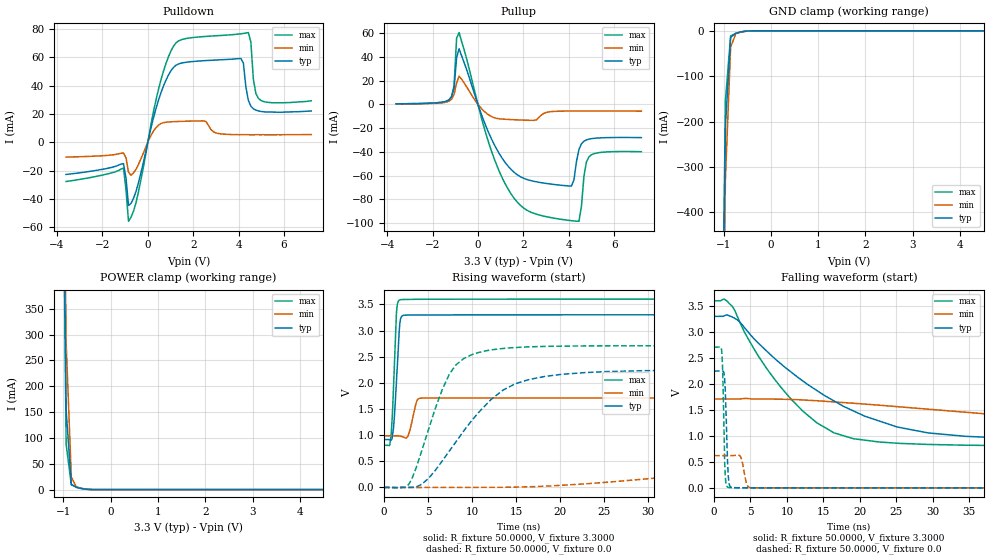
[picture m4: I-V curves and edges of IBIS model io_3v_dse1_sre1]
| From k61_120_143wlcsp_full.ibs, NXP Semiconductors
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[Model]  io_3v_dse1_sre1
|   Model io_3v_dse1_sre1
| Library cells for typ/min/max conditions are connected as defined below:
|  pad - External Pad
|  ipp_do_3v - Core Input
|  ipp_obe_3v - Output Buffer Enable
|  esd_boost - vdd_s_3v
|  esd_trigger - vss_s_3v
|  ipp_ame_3v - vss_s_3v
|  ipp_dse_3v - vdd_s_3v
|  ipp_ina_3v - NC
|  ipp_ina_mux_3v - NC
|  ipp_ind_3v - NC
|  ipp_pue_3v - vss_s_3v
|  ipp_sre_3v - vdd_s_3v
|  tie_3v - vdd_s_3v
|  tie_hi - vdd_s_lv
|  vbuf_3v - vdd_s_3v
|  vdd_s_3v - vdd_s_3v
|  vdd_s_lv - vdd_s_lv
|  vss_bulk - vss_s_3v
|  vss_s_3v - vss_s_3v
| All other pins connected to ground
Model_type I/O
Polarity   Non-Inverting
Enable   Active-High
Vinl =   1.1550V
Vinh =   2.3100V
Vmeas =  1.6500V
Cref =   25.0000pF
Rref =   50.0000
Vref =   0.0V
C_comp   1.9040pF   1.7928pF   2.1191pF
[Temperature Range]   25.0000   0.1250k   -40.0000
[Voltage Range]   3.3000V   1.7100V   3.6000V
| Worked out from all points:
|   slope of the pulldown table from 0 to 0.495 V, typ, clamps not added: 16 ohm
|   slope of the pullup table from 0 to 0.495 V, typ, clamps not added: 19.9 ohm
|   GND clamp passes 1 mA (typ) near -0.54 V on its own axis
|   POWER clamp passes 1 mA (typ) near -0.53 V on its own axis
|   rising waveform, R_fixture 50.0000, V_fixture 3.3000: 20-80 % time 474ps typ, 573ps min, 392ps max; typ from 0.916 V to 3.3 V
|   rising waveform, R_fixture 50.0000, V_fixture 0.0: 20-80 % time 6.66ns typ, 30.7ns min, 3.45ns max; typ from 0 V to 2.25 V
|   falling waveform, R_fixture 50.0000, V_fixture 3.3000: 20-80 % time 14.7ns typ, 48.4ns min, 9.12ns max; typ from 3.3 V to 0.916 V
|   falling waveform, R_fixture 50.0000, V_fixture 0.0: 20-80 % time 303ps typ, 502ps min, 251ps max; typ from 2.25 V to 0 V
[Pulldown]
|Voltage   I(typ)   I(min)   I(max)
-3.6V     -22.64mA   -10.38mA   -27.64mA
-1.07V    -15.06mA   -7.583mA   -18.14mA
-850mV    -44.54mA   -20.94mA   -55.71mA
-520mV    -34.63mA   -19mA      -42.63mA
580mV     35mA       13.27mA    44.11mA
1.46V     55.82mA    14.78mA    72.32mA
4.1V      59.16mA    5.4mA      76.58mA
4.43V     29.52mA    5.4mA      77.44mA
4.54V     25.5mA     5.3mA      70.77mA
4.65V     23.68mA    5.3mA      44.58mA
4.87V     22.2mA     5.4mA      31.08mA
7.2V      22.1mA     5.5mA      29.3mA
[Pullup]
|Voltage   I(typ)   I(min)   I(max)
-3.6V     400uA      300uA      500uA
-1.27V    3.86mA     2.75mA     3.76mA
-1.05V    14.15mA    8.34mA     15.69mA
-940mV    39.2mA     18.04mA    55.51mA
-830mV    46.74mA    23.73mA    60.38mA
1.15V     -47.61mA   -12.48mA   -64.99mA
3.13V     -66.86mA   -6.327mA   -94.95mA
4.12V     -68.7mA    -5.62mA    -97.87mA
4.45V     -37.93mA   -5.6mA     -98.38mA
4.78V     -29.93mA   -5.59mA    -48.43mA
5V        -28.86mA   -5.59mA    -42.37mA
7.2V      -27.98mA   -5.71mA    -39.85mA
[GND_clamp]
|Voltage   I(typ)   I(min)   I(max)
-3.6V     -47.78A    -47.06A    -48.3A
-1.07V    -1.101A    -1.183A    -1.105A
-960mV    -210.7mA   -326mA     -154mA
-850mV    -14.47mA   -36.11mA   -11.11mA
-740mV    -5.262mA   -6.034mA   -5.843mA
-520mV    -637uA     -915.4uA   -467.5uA
-300mV    -2.578uA   -18.09uA   -370.9nA
7.2V      0A         0A         0A
[POWER_clamp]
|Voltage   I(typ)   I(min)   I(max)
-3.6V     52.51A     51.88A     52.98A
-1.05V    1.126A     1.265A     1.065A
-940mV    154.2mA    286.1mA    88.03mA
-830mV    9.989mA    24.5mA     9.181mA
-720mV    4.227mA    4.408mA    5.116mA
-390mV    66.57uA    164uA      29.9uA
7.2V      0A         0A         0A
[Ramp]
| variable   typ   min   max
dV/dt_r  1.3478/6.6600n   0.3719/30.6544n   1.6252/3.4473n
dV/dt_f  1.4302/14.6691n   0.4336/48.3749n   1.6765/9.1203n
R_load = 50.0000
[Rising Waveform]
R_fixture= 50.0000
V_fixture= 3.3000
V_fixture_min= 1.7100
V_fixture_max= 3.6000
|time   V(typ)   V(min)   V(max)
0s        916.3mV    987.2mV    805.9mV
678.6ps   911.9mV    987.2mV    821.6mV
948.9ps   960.7mV    987.7mV    1.368V
1.44ns    2.104V     987.7mV    3.383V
1.773ns   3.082V     983.8mV    3.584V
2.015ns   3.271V     974.7mV    3.592V
2.701ns   3.295V     972.4mV    3.594V
3.727ns   3.296V     1.652V     3.597V
4.38ns    3.297V     1.708V     3.598V
250ns     3.3V       1.71V      3.6V
[Rising Waveform]
R_fixture= 50.0000
V_fixture= 0.0
V_fixture_min= 0.0
V_fixture_max= 0.0
|time   V(typ)   V(min)   V(max)
0s        2.009nV    218.2nV    1.41nV
2.888ns   -686.6uV   -1.604mV   78.44mV
5.004ns   162.9mV    -248.2uV   1.087V
6.684ns   521.6mV    -132.8uV   1.896V
8.154ns   871mV      -104.4uV   2.341V
12.1ns    1.672V     1.028mV    2.626V
14.44ns   1.941V     4.865mV    2.67V
25.46ns   2.216V     101.4mV    2.707V
79.66ns   2.246V     586.6mV    2.709V
250ns     2.246V     619.9mV    2.709V
[Falling Waveform]
R_fixture= 50.0000
V_fixture= 3.3000
V_fixture_min= 1.7100
V_fixture_max= 3.6000
|time   V(typ)   V(min)   V(max)
0s        3.3V       1.71V      3.6V
2.462ns   3.291V     1.71V      3.497V
7.003ns   2.661V     1.71V      2.34V
12.17ns   2.058V     1.692V     1.478V
16.47ns   1.673V     1.654V     1.058V
22.63ns   1.288V     1.592V     883.1mV
29.37ns   1.058V     1.514V     835.7mV
39.59ns   960.4mV    1.398V     813.8mV
91.45ns   916.7mV    1.061V     805.9mV
250ns     916.3mV    987.4mV    805.9mV
[Falling Waveform]
R_fixture= 50.0000
V_fixture= 0.0
V_fixture_min= 0.0
V_fixture_max= 0.0
|time   V(typ)   V(min)   V(max)
0s        2.246V     619.9mV    2.709V
1.03ns    2.248V     619.9mV    2.658V
1.2ns     2.248V     619.8mV    2.159V
1.392ns   2.184V     619.6mV    849.6mV
1.608ns   1.619V     619.4mV    116.7mV
1.837ns   544.9mV    619.3mV    16.25mV
2.079ns   71.93mV    619.3mV    5.402mV
3.638ns   1.828mV    602mV      1.166mV
5.279ns   845.9uV    1.196mV    674.6uV
250ns     -5.298nV   227.4nV    -4.023nV
